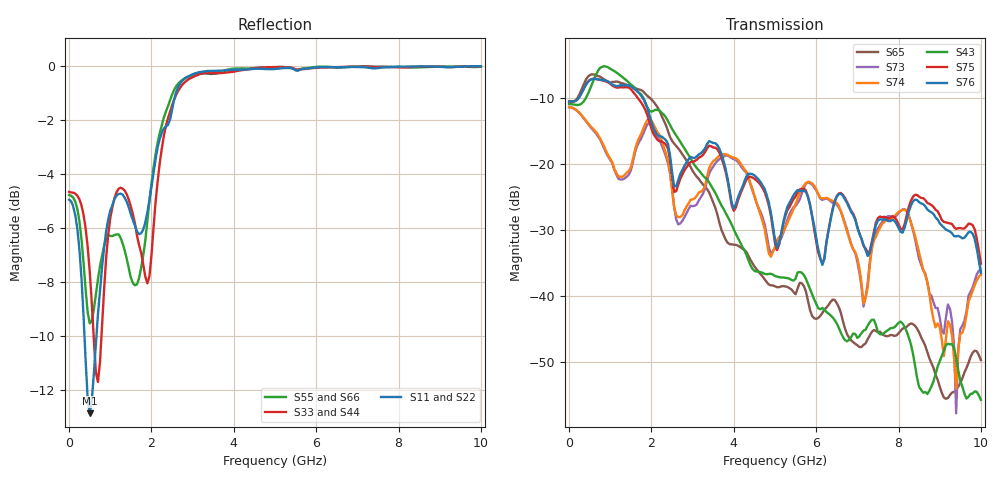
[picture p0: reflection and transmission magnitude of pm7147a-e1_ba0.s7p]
# GHz S DB R 50
! S-Parameters data
! Freq  dbS11  angS11  dbS12  angS12  dbS13  angS13  dbS14  angS14
!  dbS15  angS15  dbS16  angS16  dbS17  angS17  dbS21  angS21
!  dbS22  angS22  dbS23  angS23  dbS24  angS24  dbS25  angS25
!  dbS26  angS26  dbS27  angS27  dbS31  angS31  dbS32  angS32
!  dbS33  angS33  dbS34  angS34  dbS35  angS35  dbS36  angS36
!  dbS37  angS37  dbS41  angS41  dbS42  angS42  dbS43  angS43
!  dbS44  angS44  dbS45  angS45  dbS46  angS46  dbS47  angS47
!  dbS51  angS51  dbS52  angS52  dbS53  angS53  dbS54  angS54
!  dbS55  angS55  dbS56  angS56  dbS57  angS57  dbS61  angS61
!  dbS62  angS62  dbS63  angS63  dbS64  angS64  dbS65  angS65
!  dbS66  angS66  dbS67  angS67  dbS71  angS71  dbS72  angS72
!  dbS73  angS73  dbS74  angS74  dbS75  angS75  dbS76  angS76
!  dbS77  angS77
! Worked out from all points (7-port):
!   279 points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, 1 Hz to 10 GHz, reference 50 ohm
!   strongest paths, dB at 1 Hz, 7.943 MHz, 3.05 GHz, 6.55 GHz, 10 GHz:
!     S76: -10.6, -10.6, -19.2, -24.6, -36.5
!     S75: -10.6, -10.6, -19.6, -24.5, -35.1
!     S43: -11.0, -11.0, -20.2, -44.9, -55.8
!     S74: -11.5, -11.5, -25.3, -26.4, -36.8
!     S73: -11.5, -11.5, -26.4, -26.6, -36.1
!     S65: -10.8, -10.8, -21.6, -41.7, -49.8
!   lowest |S11| = -12.9 dB at 500 MHz (marker M1), VSWR 1.59, Z = 31.5 - j0.0742 ohm
!   |S11| at or under -10 dB: 372.7 MHz to 664.4 MHz (291.7 MHz wide, 56.3 % of centre)
